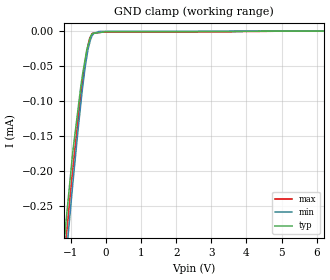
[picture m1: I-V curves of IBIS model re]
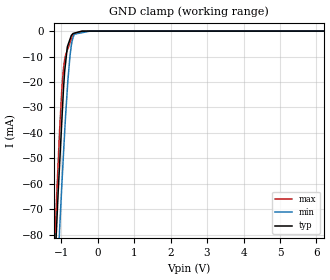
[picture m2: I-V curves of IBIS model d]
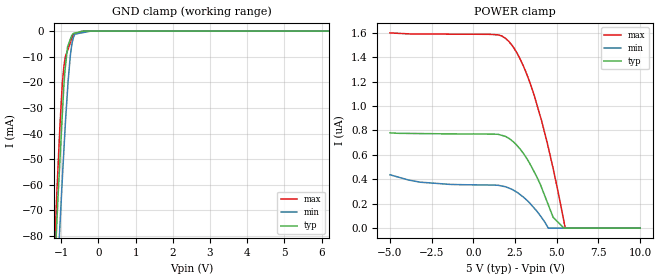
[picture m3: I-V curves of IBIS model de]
|Texas Instruments Incorporated
| Robust RS-485
| Marketing part#   Digital Voltage Range   Package-type   #pins
| SN65HVD82SOIC   4.5V - 5.5V   SOIC   8
| SN65HVD82SON   4.5V - 5.5V   SON   8
| SN65HVD82MSOP   4.5V - 5.5V   MSOP   8
[IBIS Ver]   3.2
[File name]   sn65hvd82.ibs
[File Rev]   1.0
[Date]   9/27/2012
[Source]
| Texas Instruments Incorporated.
| Analog-eLab Design Center, HPA
| 12500 TI Blvd
| Dallas, TX -75243
| e-mail: elab_scm_ibis@list.ti.com
[Notes]   Revision History:
| Rev 1.0: 9/27/2012
| - Initial version of the model
| - Model generated from simulations in TISPICE
| - Model matched to SPICE simulation
| - C_comp although listed in numerical order of value are
|   obtained from varying PVT conditions. For PVT conditions for
|   each specific value refer the buffer description under
|   respective [Model]. IBIS model user is responsible for using
|   appropriate C_comp to simulate for Signal Integrity.
| - Model names with a trailing _5 contains the model for
|   5.0V [4.5V and 5.5V].
|*  EXCEPTION:   *
|*  - For model d,there will be a leakage current in the GND clamp I-V  *
|*   Table due to a pullup transistor MP17 connected to the pad   *
|*  - For model re,there will be a leakage current in the GND clamp I-V *
|*   Table due to a pullup transistor MP17 connected to the pad   *
|*  - For model de, there will be a leakage current in the POWER   *
|*   clamp I-V Table because of the pulldown transistor connected to   *
|*   the pad.   *
|*  - For model diff_p, there will be a leakage the POWER clamp I-V Table *
|*   due to pulldown resistor on pad and the series resistor network   *
|*   connected to pad and in the GND clamp I-V Table due to resistor   *
|*  - For model diff_n, there will be a leakage the POWER clamp I-V Table *
|*   due to pulldown resistor on pad and the series resistor network   *
|*   connected to pad and in the GND clamp I-V Table due to resistor   *
|*   network connected to pad.   *
|* -  For diff_p and diff_n models,pullup non-montonicity reflects true *
|*   buffer behavior.   *
[Disclaimer]
| This model is designed as an aid for customers of Texas Instruments.
| TI and its licensors and suppliers make no warranties, either expressed
| or implied, with respect to this  model, including the warranties of
| merchantability or fitness for a particular purpose. The model is
| provided solely on an "as is" basis. The entire risk as to its quality
| and performance is with the customer.
[Copyright]
(C) Copyright 2012 Texas Instruments Incorporated.All rights reserved.
|   SN65HVD82SOIC
[Component]   SN65HVD82SOIC
[Manufacturer]   TI
[Package]   |8 SOIC   -  D package
|   typ   min   max
R_pkg   0.09289   0.05744   0.13408
L_pkg   2.53157nH   1.93942nH   3.35741nH
C_pkg   0.41401pF   0.36392pF   0.48563pF
[Pin]  signal_name   model_name   R_pin   L_pin   C_pin
1   R   r   0.06888   2.79357nH  0.48563pF
2   _RE   re   0.11765   2.52524nH  0.36564pF
3   DE   de   0.11581   2.49807nH  0.36392pF
4   D   d   0.13408   3.35741nH  0.43867pF
5   GND   gnd   0.04641   2.66825nH  0.51737pF
6   A   DIFF   0.05744   1.93942nH  0.41150pF
7   B   DIFF   0.06350   2.07574nH  0.41872pF
8   VCC   power   0.03478   2.68315nH  0.52573pF
[Diff_pin]   inv_pin   vdiff   tdelay_typ   tdelay_min   tdelay_max
6   7   0.2V   0   0   0
|   SN65HVD82SON
[Component]   SN65HVD82SON
[Manufacturer]   TI
[Package]   |8 SON -  D package
|   typ   min   max
R_pkg   0.04472   0.02919   0.06360
L_pkg   0.95638nH   0.75700nH   1.19895nH
C_pkg   0.17978pF   0.15629pF   0.20531pF
[Pin]  signal_name   model_name   R_pin   L_pin   C_pin
1   R   r   0.03112   0.84041nH  0.18584pF
2   _RE   re   0.05703   1.07068nH  0.16359pF
3   DE   de   0.05628   1.05690nH  0.16262pF
4   D   d   0.06360   1.19895nH  0.15629pF
5   GND   gnd   0.02309   0.89076nH  0.21568pF
6   A   DIFF   0.02919   0.75700nH  0.20531pF
7   B   DIFF   0.03109   0.81432nH  0.20504pF
8   VCC   power   0.01680   0.84811nH  0.21847pF
[Diff_pin]   inv_pin   vdiff   tdelay_typ   tdelay_min   tdelay_max
6   7   0.2V   0   0   0
|   SN65HVD82MSOP
[Component]   SN65HVD82MSOP
[Manufacturer]   TI
[Package]   |8 MSOP   -  D package
|   typ   min   max
R_pkg   0.04225   0.02795   0.05958
L_pkg   1.71565nH   1.51785nH   1.95887nH
C_pkg   0.41020pF   0.38033pF   0.43924pF
[Pin]  signal_name   model_name   R_pin   L_pin   C_pin
1   R   r   0.02968   1.60343nH  0.41072pF
2   _RE   re   0.05366   1.82768nH  0.39666pF
3   DE   de   0.05300   1.81461nH  0.39572pF
4   D   d   0.05958   1.95887nH  0.38033pF
5   GND   gnd   0.02230   1.65818nH  0.44110pF
6   A   DIFF   0.02795   1.51785nH  0.43924pF
7   B   DIFF   0.02961   1.57145nH  0.43851pF
8   VCC   power   0.01650   1.61542nH  0.44385pF
[Diff_pin]   inv_pin   vdiff   tdelay_typ   tdelay_min   tdelay_max
6   7   0.2V   0   0   0
|   Model Selectors
[Model Selector] DIFF
diff_p  3.3V   differential output
diff_n  3.3V   differential output
| Models and submodels in the file (6): re (Input), d (Input), de (Input), r (3-state), diff_p (I/O), diff_n (I/O)
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|   re Model
[Model]   re
Model_type   Input
Vinl = 0.8
Vinh = 2
|   typ   min   max
|   (nom PVT)   (fast PVT)   (slow PVT)
|C_comp from frequency sweep method (F=125KHz)
|Average
 C_comp   4.302e-13   4.282e-13   4.342e-13
|C_comp from LC tank measurement(L=1nH)
|Average
|Resonant Frequency(Hz)   9.999e+10   9.999e+10   9.999e+10
| C_comp   2.536e-15   2.536e-15   2.536e-15
| Where nom  PVT is Nominal Process, 5V, 27C
|   Fast PVT is Strong Process,  5.5V, -40C
|   Slow PVT is Weak Process,   4.5V, 125C
[Voltage Range]   5   4.5   5.5
|Ambient Temperature   25   85   -40
|Junction Temperature
[Temperature Range]   27   125   -40
[Power Clamp Reference]   5   4.5   5.5
[GND Clamp Reference]   0   0   0
[GND Clamp]
|   Voltage   I(typ)   I(min)   I(max)
-5V       -2.827mA   -2.634mA   -3.076mA
-1.373V   -412.5uA   -455.6uA   -424.4uA
-1.14V    -274.5uA   -327uA     -300.6uA
-1.012V   -208uA     -256.2uA   -232.5uA
-945mV    -173.2uA   -219.2uA   -198.9uA
-715mV    -78.78uA   -103.7uA   -91.44uA
-589.5mV  -39.51uA   -50.57uA   -43.43uA
-533.5mV  -24.54uA   -33.17uA   -25.36uA
-467.5mV  -12.97uA   -17.63uA   -11uA
-385mV    -3.432uA   -5.971uA   -3.243uA
-99mV     -1.492uA   -424.1nA   -1.536uA
10V       0A         0A         0A
[POWER Clamp]
|   Voltage   I(typ)   I(min)   I(max)
-5V       0A         0A         0A
-5V       0A         0A         0A
10V       0A         0A         0A
|   d Model
[Model]   d
Model_type   Input
Vinl = 0.8
Vinh = 2.0
|   typ   min   max
|   (nom PVT)   (fast PVT)   (slow PVT)
|C_comp from frequency sweep method (F=125KHz)
|Average
|C_comp   2.252e-12   2.084e-12   2.431e-12
|C_comp from LC tank measurement(L=1nH)
|Average
|Resonant Frequency(Hz)   5.830e+09   6.000e+09   5.580e+09
 C_comp   7.460e-13   7.043e-13   8.143e-13
| Where nom  PVT is Nominal Process, 5V, 27C
|   Fast PVT is Strong Process,  5.5V, -40C
|   Slow PVT is Weak Process,   4.5V, 125C
[Voltage Range]   5   4.5   5.5
|Ambient Temperature   25   85   -40
|Junction Temperature
[Temperature Range]   27   125   -40
[Power Clamp Reference]   5   4.5   5.5
[GND Clamp Reference]   0   0   0
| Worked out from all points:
|   GND clamp passes 1 mA (typ) near -0.68 V on its own axis
[GND Clamp]
|   Voltage   I(typ)   I(min)   I(max)
-5V       -1.584A    -1.507A    -1.678A
-1.238V   -115.1mA   -138.5mA   -105.3mA
-1.14V    -82mA      -108.1mA   -70.99mA
-1.122V   -76.29mA   -102.5mA   -64.65mA
-1.04V    -51.7mA    -77.46mA   -38.27mA
-935mV    -22.61mA   -48.23mA   -14.62mA
-900mV    -15.35mA   -38.86mA   -10.96mA
-814.5mV  -5.548mA   -19.39mA   -6.927mA
-751.5mV  -2.989mA   -9.075mA   -4.38mA
-670mV    -918.3uA   -2.348mA   -1.24mA
-202.5mV  -8.132uA   -612.8nA   -3.818uA
10V       0A         0A         0A
[POWER Clamp]
|   Voltage   I(typ)   I(min)   I(max)
-5V       0A         0A         0A
-4.801V   0A         0A         0A
10V       0A         0A         0A
|   de Model
[Model]   de
Model_type   Input
Vinl = 0.8
Vinh = 2
|   typ   min   max
|   (nom PVT)   (fast PVT)   (slow PVT)
|C_comp from frequency sweep method (F=125KHz)
|Average
|C_comp   2.259e-12   2.100e-12   2.427e-12
|C_comp from LC tank measurement(L=1nH)
|Average
|Resonant Frequency(Hz)   5.830e+09   6.000e+09   5.580e+09
 C_comp   7.460e-13   7.043e-13   8.143e-13
| Where nom  PVT is Nominal Process, 5V, 27C
|   Fast PVT is Strong Process,  5.5V, -40C
|   Slow PVT is Weak Process,   4.5V, 125C
[Voltage Range]   5   4.5   5.5
|Ambient Temperature   25   85   -40
|Junction Temperature
[Temperature Range]   27   125   -40
[Power Clamp Reference]   5   4.5   5.5
[GND Clamp Reference]   0   0   0
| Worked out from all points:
|   GND clamp passes 1 mA (typ) near -0.68 V on its own axis
[GND Clamp]
|   Voltage   I(typ)   I(min)   I(max)
-5V       -1.575A    -1.498A    -1.669A
-1.238V   -114.5mA   -137.6mA   -104.9mA
-1.14V    -81.57mA   -107.5mA   -70.7mA
-1.122V   -75.9mA    -101.9mA   -64.39mA
-1.04V    -51.45mA   -77.02mA   -38.16mA
-935mV    -22.54mA   -47.98mA   -14.62mA
-900mV    -15.32mA   -38.67mA   -10.96mA
-814.5mV  -5.545mA   -19.31mA   -6.927mA
-751.5mV  -2.988mA   -9.051mA   -4.38mA
-670mV    -918.3uA   -2.345mA   -1.24mA
-202.5mV  -7.903uA   -499.5nA   -3.375uA
10V       0A         0A         0A
[POWER Clamp]
|   Voltage   I(typ)   I(min)   I(max)
-5V       780.2nA    437.2nA    1.599uA
-3.177V   774.5nA    376.3nA    1.59uA
968mV     770.1nA    353.2nA    1.587uA
1.925V    751.2nA    339.1nA    1.554uA
2.36V     711.4nA    314.3nA    1.489uA
2.794V    648.6nA    275.7nA    1.388uA
3.217V    566.5nA    227.5nA    1.255uA
3.652V    459.4nA    163.1nA    1.084uA
4.487V    192.3nA    0A         663.8nA
4.785V    87.54nA    0A         486.8nA
5.505V    0A         0A         0A
10V       0A         0A         0A
